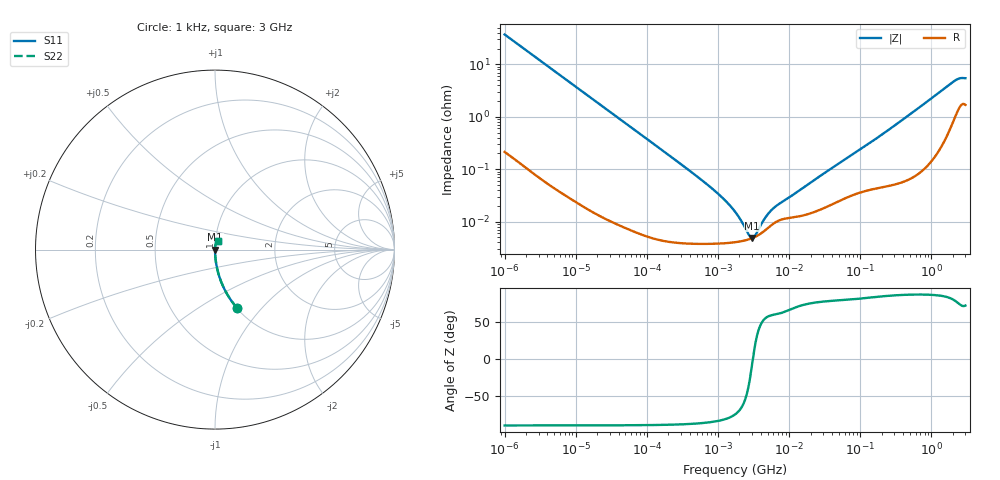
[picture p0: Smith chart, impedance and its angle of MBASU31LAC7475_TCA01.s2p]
! MBASU31LAC7475_TCA01  S-PARAMETER MODEL  ( Standard Model )
! Model Generated by TAIYO YUDEN Corporation (http://www.ty-top.com)
! Version 1.0
! TAIYO YUDEN Control No. 220601
! Copyright(c) 2016 TAIYO YUDEN CO.,LTD. All Rights Reserved.
! Product Description (link to TY-COMPAS)
! https://ds.yuden.co.jp/TYCOMPAS/or/detail?pn=MBASU31LAC7475KTCA01&u=M
! Products Name : Multilayer Ceramic Capacitors
! Characteristics :
!  Capacitance : 4.7 [uF] , Rated Voltage : 50 [V] , TCC : X7S
!  Case Size : 3.2 x 1.6 / 0.126 x 0.063 [mm/inch] , Thickness : 1.6 / 0.063 [mm/inch]
!  (Conditions: Temperature = 25 [degC] , DC Bias Voltage = 0 [V])
! External Node Assignments :
!  1  o---| |---o  2
! GND o---------o GND
! Frequency Range : 1kHz  -  3GHz  [ 401 STEP ]
# MHZ S RI R 50
! Freq[MHz].  S11 Real  S11 Imag  S21 Real  S21 Imag  S12 Real  S12 Imag  S22 Real  S22 Imag
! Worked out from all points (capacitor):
!   401 points, 1 kHz to 3 GHz, reference 50 ohm
!   read as one part in series: C = 4.27 uF near 1.077 kHz
!   lowest |Z| = 4.87 mohm at 3.03 MHz (marker M1)
!   series resonance near 3.091 MHz, so ESL is about 620 pH
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0.001  0.1231 -0.3257  0.8769 0.3257  0.8769 0.3257  0.1231 -0.3257
0.001685  0.0478 -0.2105  0.9522 0.2105  0.9522 0.2105  0.0478 -0.2105
0.00306  0.0154 -0.1202  0.9846 0.1202  0.9846 0.1202  0.0154 -0.1202
0.005768  0.00457 -0.0646  0.9954 0.0646  0.9954 0.0646  0.00457 -0.0646
0.01216  0.00115 -0.0308  0.9988 0.0308  0.9988 0.0308  0.00115 -0.0308
0.147855  5.12e-05 -0.00256  0.9999 0.00256  0.9999 0.00256  5.12e-05 -0.00256
0.419985  3.87e-05 -0.000886  1 0.000886  1 0.000886  3.87e-05 -0.000886
0.791611  3.79e-05 -0.000447  1 0.000447  1 0.000447  3.79e-05 -0.000447
1.238299  3.88e-05 -0.000257  1 0.000257  1 0.000257  3.88e-05 -0.000257
1.732051  4.05e-05 -0.00015  1 0.00015  1 0.00015  4.05e-05 -0.00015
2.087011  4.21e-05 -9.88e-05  1 9.88e-05  1 9.88e-05  4.21e-05 -9.88e-05
2.24859  4.3e-05 -7.93e-05  1 7.93e-05  1 7.93e-05  4.3e-05 -7.93e-05
3.03007  4.85e-05 -4.85e-06  1 4.85e-06  1 4.85e-06  4.85e-05 -4.85e-06
3.93371  5.84e-05 5.88e-05  0.9999 -5.88e-05  0.9999 -5.88e-05  5.84e-05 5.88e-05
4.238263  6.27e-05 7.69e-05  0.9999 -7.69e-05  0.9999 -7.69e-05  6.27e-05 7.69e-05
5.502215  8.35e-05 0.000137  0.9999 -0.000137  0.9999 -0.000137  8.35e-05 0.000137
6.387174  9.67e-05 0.000167  0.9999 -0.000167  0.9999 -0.000167  9.67e-05 0.000167
21.06097  0.000148 0.000565  0.9999 -0.000565  0.9999 -0.000565  0.000148 0.000565
256.0921  0.000515 0.00575  0.9995 -0.00575  0.9995 -0.00575  0.000515 0.00575
1990.675  0.00963 0.0445  0.9904 -0.0445  0.9904 -0.0445  0.00963 0.0445
2398.636  0.0162 0.0499  0.9838 -0.0499  0.9838 -0.0499  0.0162 0.0499
3000  0.0191 0.0501  0.9809 -0.0501  0.9809 -0.0501  0.0191 0.0501
